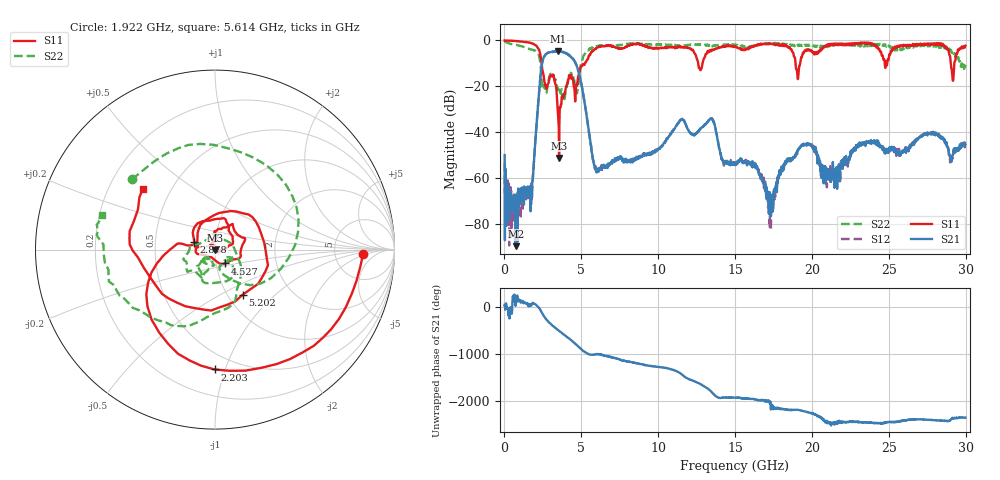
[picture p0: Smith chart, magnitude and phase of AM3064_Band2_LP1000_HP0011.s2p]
# Hz S DB R 50.0
!freq dBS11 angS11 dBS21 angS21 dBS12 angS12 dBS22 angS22
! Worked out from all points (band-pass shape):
!   1600 points, 10 MHz to 29.98 GHz, reference 50 ohm
!   highest |S21| = -4.67 dB at 3.478 GHz (marker M1); lowest = -89.5 dB at 759.8 MHz (marker M2)
!   |S21| within 3 dB of the highest: 2.539 GHz to 4.403 GHz (1.864 GHz wide, 53.7 % of centre)
!   lowest |S11| = -51.1 dB at 3.553 GHz (marker M3), VSWR 1.01, Z = 50.1 - j0.274 ohm
!   |S11| at or under -10 dB: 2.416 GHz to 5.243 GHz (2.827 GHz wide, 73.8 % of centre); 12.6 GHz to 12.88 GHz (282.8 MHz wide, 2.22 % of centre); 18.93 GHz to 19.23 GHz (301.6 MHz wide, 1.58 % of centre)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
!   |S22| runs from -25.5 to -0.2 dB; largest |S21 - S12| = 0.018
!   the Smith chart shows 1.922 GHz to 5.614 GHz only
!   S11 on the Smith chart (normalised r, x): 1.922 GHz: 10, -1; 2.203 GHz: 0.38, -0.92; 2.878 GHz: 0.79, +0.07; 4.527 GHz: 1.11, -0.17; 5.202 GHz: 1.17, -0.64; 5.614 GHz: 0.35, +0.33
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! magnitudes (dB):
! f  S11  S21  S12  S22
! 10 MHz  0.0  -49.9  -53.3  -0.2
! 759.8 MHz  -0.3  -89.5  -69.4  -2.0
! 1.659 GHz  -1.0  -65.4  -63.7  -3.8
! 1.922 GHz  -1.7  -52.3  -53.1  -4.4
! 2.203 GHz  -3.5  -26.6  -26.6  -5.8
! 2.878 GHz  -18.2  -5.3  -5.3  -17.3
! 3.478 GHz  -31.8  -4.7  -4.8  -21.3
! 3.553 GHz  -51.1  -4.9  -4.7  -20.6
! 4.527 GHz  -20.4  -8.7  -8.6  -17.0
! 5.015 GHz  -11.2  -19.3  -19.4  -9.5
! 5.202 GHz  -10.6  -26.6  -26.6  -6.2
! 5.614 GHz  -5.6  -45.8  -45.2  -3.7
! 6.102 GHz  -2.9  -56.0  -57.6  -2.4
! 10 GHz  -3.4  -47.1  -47.3  -1.8
! 13.43 GHz  -4.5  -33.9  -33.9  -2.4
! 15 GHz  -2.5  -54.3  -53.5  -1.9
! 16.3 GHz  -2.1  -55.2  -54.6  -2.2
! 17.29 GHz  -1.5  -72.7  -68.1  -1.3
! 19.99 GHz  -4.5  -46.2  -45.9  -2.0
! 20.93 GHz  -2.3  -55.4  -59.1  -2.1
! 25 GHz  -7.9  -47.2  -48.4  -2.2
! 29.98 GHz  -2.3  -45.3  -44.9  -10.5
